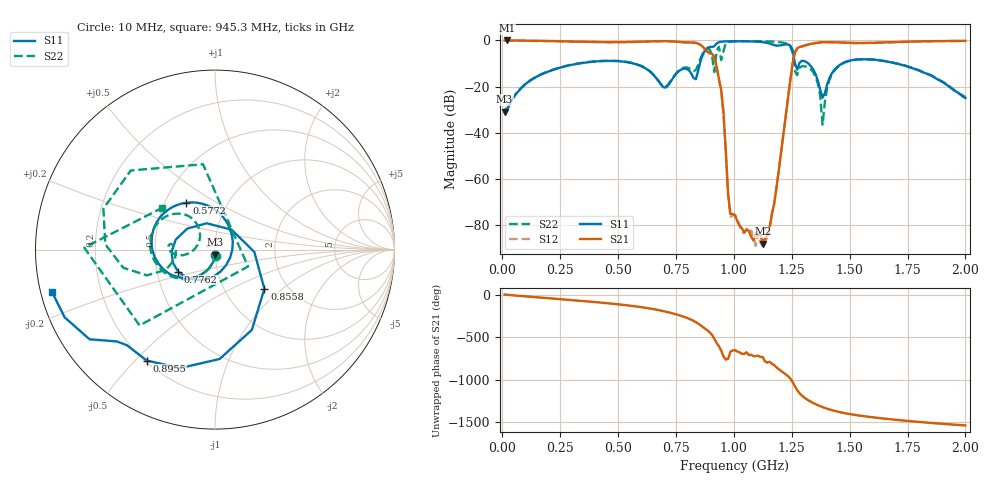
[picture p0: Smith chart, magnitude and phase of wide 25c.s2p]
!Agilent Technologies,E8363B,SG43030131,A.07.50.48
!Agilent E8363B: A.07.50.48
!Date: Monday, December 01, 2025 21:14:28
!Correction: S11(Full 2 Port(1,2))
!S21(Full 2 Port(1,2))
!S12(Full 2 Port(1,2))
!S22(Full 2 Port(1,2))
!S2P File: Measurements: S11, S21, S12, S22:
# Hz S  dB  R 50
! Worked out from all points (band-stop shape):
!   201 points, 10 MHz to 2 GHz, reference 50 ohm
!   highest |S21| = 0.00 dB at 19.95 MHz (marker M1); lowest = -88.1 dB at 1.124 GHz (marker M2)
!   |S21| within 3 dB of the highest: start of sweep to 868.2 MHz; 1.281 GHz to end of sweep
!   lowest |S11| = -30.8 dB at 10 MHz (marker M3), VSWR 1.06, Z = 50.1 - j2.89 ohm
!   |S11| at or under -10 dB: start of sweep to 331.5 MHz; 567 MHz to 853.5 MHz (286.6 MHz wide, 40.3 % of centre); 1.701 GHz to end of sweep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
!   |S22| runs from -36.5 to -0.3 dB; largest |S21 - S12| = 0.033
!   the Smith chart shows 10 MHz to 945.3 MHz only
!   S11 on the Smith chart (normalised r, x): 10 MHz: 1.00, -0.06; 577.1 MHz: 0.64, +0.37; 776.1 MHz: 0.64, -0.17; 855.8 MHz: 1.53, -0.76; 895.5 MHz: 0.21, -0.54; 945.3 MHz: 0.03, -0.13
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1e7  -30.80 -85.9  -0.03 -0.3  -0.06 -2.1  -29.48 -82.0
1.995e7  -30.21 -87.7  0.00 -3.1  -0.06 -4.6  -29.81 -90.3
3.483e8  -9.74 -166.9  -0.56 -76.2  -0.64 -76.3  -9.65 -163.5
5.7715e8  -10.29 121.3  -0.58 -139.6  -0.67 -139.8  -10.21 140.2
6.7665e8  -17.94 42.8  -0.29 175.9  -0.37 175.7  -17.68 130.4
7.7615e8  -12.42 -149.2  -0.71 106.0  -0.79 105.8  -12.07 -177.8
8.5575e8  -9.09 -38.5  -1.87 -0.5  -1.96 -0.8  -7.84 -159.3
8.9555e8  -2.78 -121.6  -5.53 -82.9  -5.61 -83.2  -3.82 136.8
9.254e8  -1.32 -144.4  -11.19 151.8  -11.28 151.5  -4.49 -134.8
9.453e8  -0.56 -165.3  -21.40 62.8  -21.46 62.4  -8.49 142.1
9.851e8  -0.35 165.6  -75.23 48.0  -76.38 46.2  -0.47 157.9
1.005e9  -0.35 153.4  -75.72 66.2  -75.42 60.9  -0.36 142.6
1.1244e9  -0.73 63.4  -88.07 -14.3  -89.13 -60.0  -0.34 78.3
1.1841e9  -2.26 -75.1  -63.69 -135.5  -64.29 -137.6  -0.58 36.3
1.2239e9  -1.71 168.7  -32.67 142.1  -32.77 141.8  -1.24 -12.7
1.2637e9  -9.86 77.7  -5.19 1.6  -5.30 1.5  -13.23 -122.2
1.29355e9  -8.82 111.1  -2.54 -107.3  -2.61 -107.4  -11.20 -144.8
1.3433e9  -12.64 73.4  -1.27 163.6  -1.35 163.4  -13.79 80.6
1.3831e9  -24.78 108.0  -0.75 116.4  -0.83 116.2  -36.52 -32.5
1.4428e9  -11.80 152.5  -0.84 66.9  -0.91 66.8  -12.09 153.1
1.67165e9  -9.32 77.3  -0.78 -25.1  -0.85 -25.4  -9.26 50.5
2e9  -24.99 66.2  -0.16 -99.2  -0.23 -99.4  -24.66 -83.9
